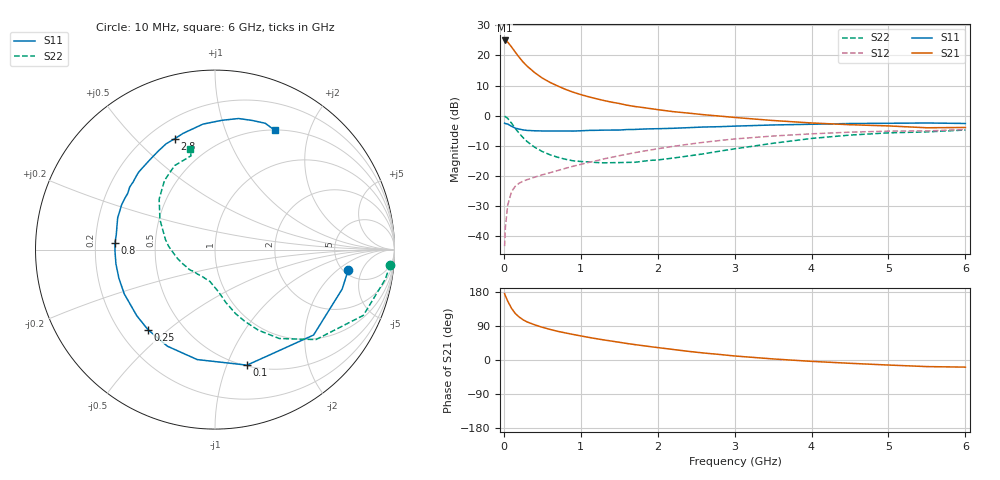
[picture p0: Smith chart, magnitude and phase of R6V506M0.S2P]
! SIEMENS Small Signal Semiconductors
! BFR193
! Si NPN RF Bipolar Junction Transistor in SOT23
! VCE = 0.5 V  IC = 6 mA
! Common Emitter S-Parameters:  May  1996
# GHz  S  MA  R  50
!  f  S11  S21  S12  S22
! GHz  MAG  ANG  MAG  ANG  MAG  ANG  MAG  ANG
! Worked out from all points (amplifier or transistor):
!   36 points, 10 MHz to 6 GHz, reference 50 ohm
!   highest |S21| = 24.9 dB at 10 MHz (marker M1)
!   |S21| within 3 dB of that: start of sweep to 124.3 MHz
!   unconditionally stable (mu >= 1): 788.9 MHz to 2.456 GHz; 5.437 GHz to end of sweep
!   at 250 MHz: K = 0.49, MSG = 19.7 dB, |S12| = -21.7 dB
!   at 1.4 GHz: K = 1.08, MAG = 7.4 dB, |S12| = -13.8 dB
!   at 6 GHz: K = 1.00, MAG = 0.1 dB, |S12| = -4.6 dB
!   S11 on the Smith chart (normalised r, x): 10 MHz: 5.56, -2.84; 100 MHz: 0.51, -1.18; 250 MHz: 0.32, -0.43; 800 MHz: 0.28, +0.03; 2.8 GHz: 0.30, +0.66; 6 GHz: 0.51, +1.50
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0.01  0.7516 -8.5  17.63 175.1  0.0069 84.4  0.9805 -5.0
0.02  0.7417 -17.3  17.62 169.6  0.014 81.6  0.9628 -9.9
0.05  0.7268 -40.9  16.57 155.4  0.033 70.3  0.9043 -23.9
0.1  0.668 -74.5  13.79 136.4  0.0555 57.2  0.7535 -41.7
0.15  0.6207 -99.2  11.23 122.4  0.068 49.2  0.6118 -54.1
0.2  0.6 -116.2  9.259 113.3  0.0763 45.1  0.5103 -61.7
0.25  0.5818 -129.9  7.755 106.1  0.0825 43.1  0.4332 -67.4
0.3  0.5708 -139.7  6.668 100.7  0.087 42.5  0.3756 -72.1
0.4  0.5626 -154.0  5.178 92.9  0.0958 43.1  0.3009 -78.4
0.5  0.5587 -163.5  4.201 86.4  0.1049 44.1  0.2549 -82.8
0.6  0.5577 -171.8  3.562 80.8  0.1136 45.8  0.2252 -87.1
0.8  0.5587 176.3  2.734 71.5  0.1342 48.6  0.1898 -95.6
0.9  0.5563 171.3  2.452 67.4  0.1455 49.6  0.179 -99.3
1.1  0.5704 161.9  2.061 59.8  0.1678 50.5  0.1716 -107.1
1.3  0.5771 154.3  1.785 53.0  0.1926 50.7  0.1657 -115.7
1.6  0.5895 143.7  1.494 43.6  0.2301 49.8  0.1684 -130.2
2.2  0.6185 125.8  1.167 27.8  0.3105 44.6  0.1986 -157.5
2.8  0.6574 109.9  0.987 14.7  0.3875 36.6  0.2582 176.2
3.5  0.7023 95.5  0.832 2.8  0.4607 25.4  0.3495 151.4
4.5  0.742 79.8  0.709 -8.7  0.5335 10.6  0.4774 126.1
5.5  0.7575 68.3  0.631 -17.4  0.5589 -3.4  0.5393 104.3
6  0.7431 63.3  0.638 -18.8  0.5906 -7.6  0.5791 104.0
